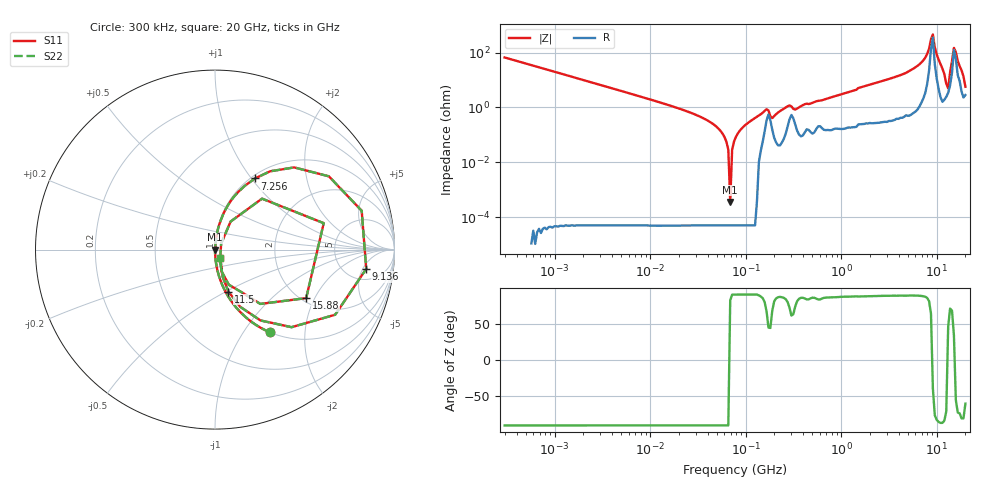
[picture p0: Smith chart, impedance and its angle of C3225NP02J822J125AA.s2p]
! S-parameter Generated by TDK Corporation
! Copyright(C) 2015 TDK Corporation.
! All Rights Reserved.
! TDK P/N: C3225NP02J822J125AA (Multilayer Ceramic Chip Capacitors)
! Property: C=8.2nF
! Size(LxWxT): 3.2x2.5x1.25mm, 0.126x0.098x0.049inches
! Model Type: s2p (Touchstone File Format Version 1.0)
! Frequency: DC=Yes Start=0.3MHz Stop=20000MHz 243points Log-sweep
! Note:
! Model Generated on Jun. 23, 2015
! Hash(MD5):
! Port Assignments:
!  1 ---| |--- 2
! Applicable Conditions:
!  Temperature = 25 degC
!  DC Bias Voltage = 0 V
!  Small Signal Operation
! Terms and conditions regarding TDK Simulation Models
! (1)This simulation model is being provided solely for informational purposes. Please refer to the specifications of the products in terms of detailed characteristics of such products.
! (2)In no event shall TDK Corporation of any of its subsidiaries be liable for any loss or damage arising, directly or indirectly,
!  From any information contained in this simulation model, including, but not limited to loss or damages arising from any inaccuracies, omissions or errors in connection with such information.
! (3)Any and all copyrights on this simulation model are owned by TDK Corporation.
!  Duplication or redistribution of this simulation model without prior written permission from TDK Corporation is prohibited.
! (4)This simulation model is subject to any modification or change without any prior notice.
! (5)Neither TDK Corporation nor any of its subsidiaries shall make any warranty, express or implied,
!  Including but not limited to the correctness, implied warranties of merchantability and fitness for a particular purpose with respect to this simulation models.
! (6)The use of this simulation model shall be deemed to have consented to the terms and conditions hereof.
# MHz S MA R 50
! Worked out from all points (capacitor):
!   242 points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, 300 kHz to 20 GHz, reference 50 ohm
!   read as one part in series: C = 8.01 nF near 314.2 kHz
!   lowest |Z| = 357 uohm at 69.03 MHz (marker M1)
!   series resonance near 68.99 MHz, so ESL is about 660 pH
!   S11 on the Smith chart (normalised r, x): 300 kHz: 1.00, -1.32; 7.256 GHz: 1.04, +1.04; 9.136 GHz: 7.67, -5.92; 11.5 GHz: 1.03, -0.51; 15.88 GHz: 2.12, -1.72; 20 GHz: 1.06, -0.10
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0.3  0.5512 -56.6  0.8344 33.4  0.8344 33.4  0.5512 -56.6
1.985118  0.09986 -84.3  0.995 5.7  0.995 5.7  0.09986 -84.3
12.54397  0.01537 -89.4  0.9998 0.9  0.9998 0.9  0.01537 -89.4
47.74252  0.002206 -92.6  0.9999 0.1  0.9999 0.1  0.002206 -92.6
60.11549  0.0008359 -96.8  0.9999 0.0  0.9999 0.0  0.0008359 -96.8
69.02956  0.0001409 178.7  0.9999 -0.0  0.9999 -0.0  0.0001409 178.7
79.26541  0.0008579 97.9  0.9999 -0.0  0.9999 -0.0  0.0008579 97.9
165.7079  0.008537 66.5  0.9966 -0.4  0.9966 -0.4  0.008537 66.5
190.2795  0.004072 67.7  0.9985 -0.2  0.9985 -0.2  0.004072 67.7
288.0964  0.01177 71.4  0.9963 -0.6  0.9963 -0.6  0.01177 71.4
500.8786  0.01463 84.8  0.9988 -0.8  0.9988 -0.8  0.01463 84.8
3165.055  0.1076 82.1  0.991 -6.2  0.991 -6.2  0.1076 82.1
7255.597  0.4544 60.7  0.8723 -27.0  0.8723 -27.0  0.4544 60.7
8331.474  0.7545 32.8  0.546 -48.2  0.546 -48.2  0.7545 32.8
9135.962  0.8494 -7.3  0.1861 32.2  0.1861 32.2  0.8494 -7.3
10018.13  0.6074 -45.4  0.7174 37.0  0.7174 37.0  0.6074 -45.4
11503.64  0.246 -72.2  0.9541 14.2  0.9541 14.2  0.246 -72.2
13209.43  0.0475 43.9  0.9663 -2.0  0.9663 -2.0  0.0475 43.9
14484.93  0.3864 47.3  0.7846 -20.9  0.7846 -20.9  0.3864 47.3
15168.15  0.6233 13.7  0.4205 -20.3  0.4205 -20.3  0.6233 13.7
15883.6  0.5755 -28.0  0.5531 27.2  0.5531 27.2  0.5755 -28.0
20000  0.05497 -57.2  0.9713 2.7  0.9713 2.7  0.05497 -57.2
